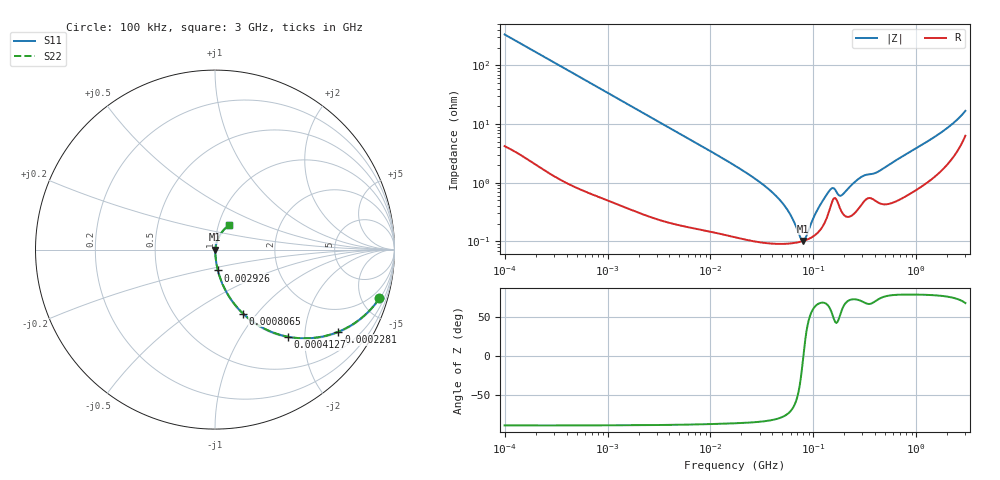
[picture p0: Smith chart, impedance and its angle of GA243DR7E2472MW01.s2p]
!Murata Part Number: GA243DR7E2472MW01
!These Parameters are Measured in Series Mode Connection
!Data Generated on Jun 19, 2026
!  o--ll--o
!Port1  Port2
!  o------o
!Operation Temp=25[degC], DC Bias Voltage=0[V]
!Freq. Start=100[kHz] Stop=3[GHz] 401[Steps]
# Hz S RI R 50
!Freq.(Hz) S11(Real) S11(Imag) S21(Real) S21(Imag) S12(Real) S12(Imag) S22(Real) S22(Imag)
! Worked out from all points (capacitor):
!   401 points, 100 kHz to 3 GHz, reference 50 ohm
!   read as one part in series: C = 4.7 nF near 105.3 kHz
!   lowest |Z| = 102 mohm at 79.24 MHz (marker M1)
!   series resonance near 79.98 MHz, so ESL is about 840 pH
!   S11 on the Smith chart (normalised r, x): 100 kHz: 1.08, -6.75; 228.1 kHz: 1.04, -2.98; 412.7 kHz: 1.02, -1.65; 806.5 kHz: 1.01, -0.85; 2.926 MHz: 1.00, -0.24; 3 GHz: 1.13, +0.31
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100000  0.9165 -0.2705  0.0835 0.2705  0.0835 0.2705  0.9165 -0.2705
228123  0.6877 -0.4576  0.3123 0.4576  0.3123 0.4576  0.6877 -0.4576
412671  0.4072 -0.4855  0.5928 0.4855  0.5928 0.4855  0.4072 -0.4855
562235  0.2724 -0.4391  0.7276 0.4391  0.7276 0.4391  0.2724 -0.4391
806524  0.1563 -0.3564  0.8437 0.3564  0.8437 0.3564  0.1563 -0.3564
2925885  0.0161 -0.116  0.9839 0.116  0.9839 0.116  0.0161 -0.116
3161081  0.0141 -0.1076  0.9859 0.1076  0.9859 0.1076  0.0141 -0.1076
1.77727e7  0.00152 -0.0189  0.9985 0.0189  0.9985 0.0189  0.00152 -0.0189
3.13325e7  0.00105 -0.00969  0.9989 0.00969  0.9989 0.00969  0.00105 -0.00969
4.611977e7  0.000934 -0.00525  0.9991 0.00525  0.9991 0.00525  0.000934 -0.00525
5.815973e7  0.000928 -0.00296  0.9991 0.00296  0.9991 0.00296  0.000928 -0.00296
7.525761e7  0.000989 -0.000566  0.999 0.000566  0.999 0.000566  0.000989 -0.000566
7.923846e7  0.00101 -8.66e-05  0.999 8.66e-05  0.999 8.66e-05  0.00101 -8.66e-05
8.560801e7  0.00106 0.000643  0.9989 -0.000643  0.9989 -0.000643  0.00106 0.000643
9.738194e7  0.00119 0.00191  0.9988 -0.00191  0.9988 -0.00191  0.00119 0.00191
1.166348e8  0.00158 0.00389  0.9984 -0.00389  0.9984 -0.00389  0.00158 0.00389
1.470833e8  0.00399 0.0066  0.996 -0.0066  0.996 -0.0066  0.00399 0.0066
1.854806e8  0.00339 0.00497  0.9966 -0.00497  0.9966 -0.00497  0.00339 0.00497
2.874592e8  0.00414 0.0116  0.9959 -0.0116  0.9959 -0.0116  0.00414 0.0116
5.475153e8  0.00476 0.0198  0.9952 -0.0198  0.9952 -0.0198  0.00476 0.0198
1.701687e9  0.0194 0.0659  0.9806 -0.0659  0.9806 -0.0659  0.0194 0.0659
3e9  0.0794 0.1352  0.9206 -0.1352  0.9206 -0.1352  0.0794 0.1352
